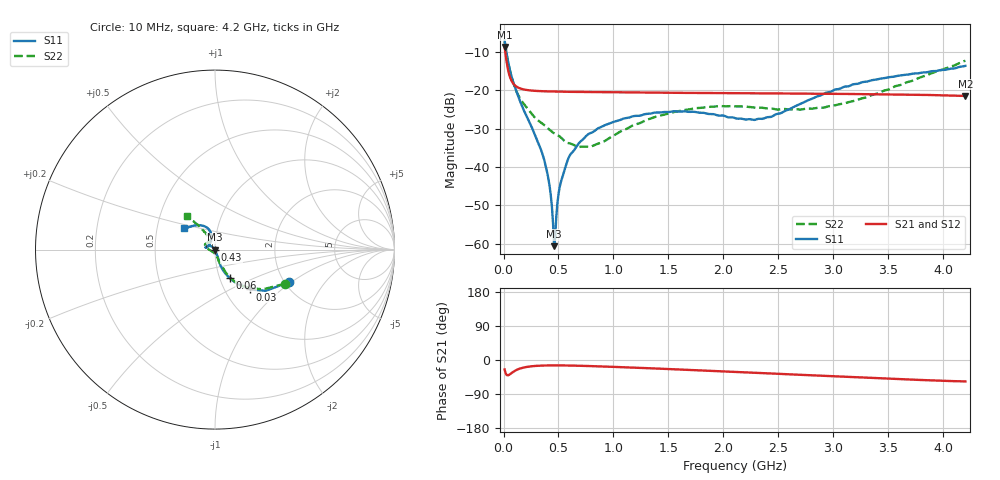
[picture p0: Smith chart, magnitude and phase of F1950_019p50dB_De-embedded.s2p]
! Integrated Device Technology
! Corporate Headquarters
! 6024 Silver Creek Valley Road
! San Jose, CA 95138  USA
! Phone:  1-408-284-8200
! Toll Free:  1-800-223-1366
! Webpage:  http://www.idt.com/
! Timing and RF Division
! 515 Groton Road, Suite 102
! Westford, MA 01886-6024
! Device:  F1950
! Description: 7-bit 0.25 dB Digital Step Attenuator
! Frequency:  150.0 -  4000.00 MHz
! Package:  4x4 mm Thin QFN Plastic Package: 24 pin
! Ports:  2 RF, 12 DC
!  Pin  1  = D0
!  Pin  2  = VDD
!  Pin  3  = Vmode
!  Pin  4  = GND
!  Pin  5  = RF1  =  Port 1
!  Pin  6  = GND
!  Pin  7  = GND
!  Pin  8  = GND
!  Pin  9  = GND
!  Pin 10  = GND
!  Pin 11  = GND
!  Pin 12  = GND
!  Pin 13  = GND
!  Pin 14  = RF2  =  Port 2
!  Pin 15  = GND
!  Pin 16  = LE
!  Pin 17  = CLK
!  Pin 18  = DATE
!  Pin 19  = D6
!  Pin 20  = D5
!  Pin 21  = D4
!  Pin 22  = D3
!  Pin 23  = D2
!  Pin 24  = D1
! State:  78
! Atten State:  19.50 dB
! Voltage:  +5.00 Volts
! Current:  Not Measured mA
! Data:  The device was measured on a the F195X evaluation board which has
!  individual transmission lines to the RF pins.  Data was collected
!  using a calibrated network analyzer.  The evaluation board was
!  de-embedded using a TRL calibration technique.
!  The reference plane is the edge of the package pin.
! Misc:  Board 2019
!  Action Tracker AT0250
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# GHz S dB R 50
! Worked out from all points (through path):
!   420 points, 10 MHz to 4.2 GHz, reference 50 ohm
!   highest |S21| = -8.63 dB at 10 MHz (marker M1); lowest = -21.4 dB at 4.2 GHz (marker M2)
!   group delay of S21, straight-line fit = 29.1 ps
!   lowest |S11| = -60.7 dB at 460 MHz (marker M3), VSWR 1.00, Z = 49.9 - j0.073 ohm
!   |S11| at or under -10 dB: 26.82 MHz to end of sweep
!   |S22| runs from -34.8 to -7.2 dB; largest |S21 - S12| = 0.00016
!   S11 on the Smith chart (normalised r, x): 10 MHz: 2.10, -0.96; 30 MHz: 1.31, -0.64; 60 MHz: 1.12, -0.37; 430 MHz: 1.00, -0.01; 4.2 GHz: 0.69, +0.17
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0.01  -6.95 -23.9  -8.63 -25.0  -8.63 -25.0  -7.23 -25.9
0.03  -10.57 -48.5  -12.83 -39.8  -12.83 -39.8  -10.93 -48.7
0.06  -14.96 -62.6  -16.59 -37.4  -16.59 -37.4  -15.00 -61.6
0.15  -22.78 -71.5  -19.47 -22.6  -19.47 -22.6  -22.06 -69.9
0.35  -36.26 -67.1  -20.20 -14.7  -20.20 -14.7  -28.56 -77.0
0.4  -41.84 -68.6  -20.25 -14.4  -20.25 -14.4  -29.76 -77.9
0.43  -47.41 -75.4  -20.28 -14.2  -20.28 -14.3  -30.54 -80.0
0.45  -54.54 -89.1  -20.29 -14.2  -20.29 -14.2  -31.02 -82.6
0.46  -60.68 -127.8  -20.30 -14.2  -20.30 -14.2  -31.21 -83.9
0.48  -52.95 142.3  -20.31 -14.2  -20.31 -14.2  -31.52 -86.3
0.51  -45.35 135.2  -20.32 -14.2  -20.32 -14.2  -32.00 -88.4
0.57  -39.36 131.6  -20.35 -14.5  -20.35 -14.5  -33.55 -95.9
0.61  -36.66 134.1  -20.37 -14.7  -20.37 -14.7  -33.90 -103.1
0.71  -33.10 136.2  -20.40 -15.4  -20.40 -15.4  -34.72 -120.7
0.99  -28.34 146.4  -20.49 -18.0  -20.49 -18.0  -31.97 -167.6
1.41  -25.77 162.5  -20.60 -22.7  -20.60 -22.7  -26.66 168.3
1.73  -25.58 168.0  -20.65 -26.5  -20.65 -26.6  -24.70 159.2
2.11  -27.27 157.2  -20.72 -31.5  -20.72 -31.5  -24.18 150.0
2.43  -26.92 124.8  -20.78 -35.5  -20.78 -35.5  -24.74 140.5
2.81  -22.13 104.2  -20.85 -40.6  -20.85 -40.6  -24.76 125.9
3.51  -16.52 116.8  -21.04 -49.5  -21.03 -49.6  -19.67 119.6
4.2  -13.58 145.7  -21.44 -56.5  -21.44 -56.6  -12.23 129.9
